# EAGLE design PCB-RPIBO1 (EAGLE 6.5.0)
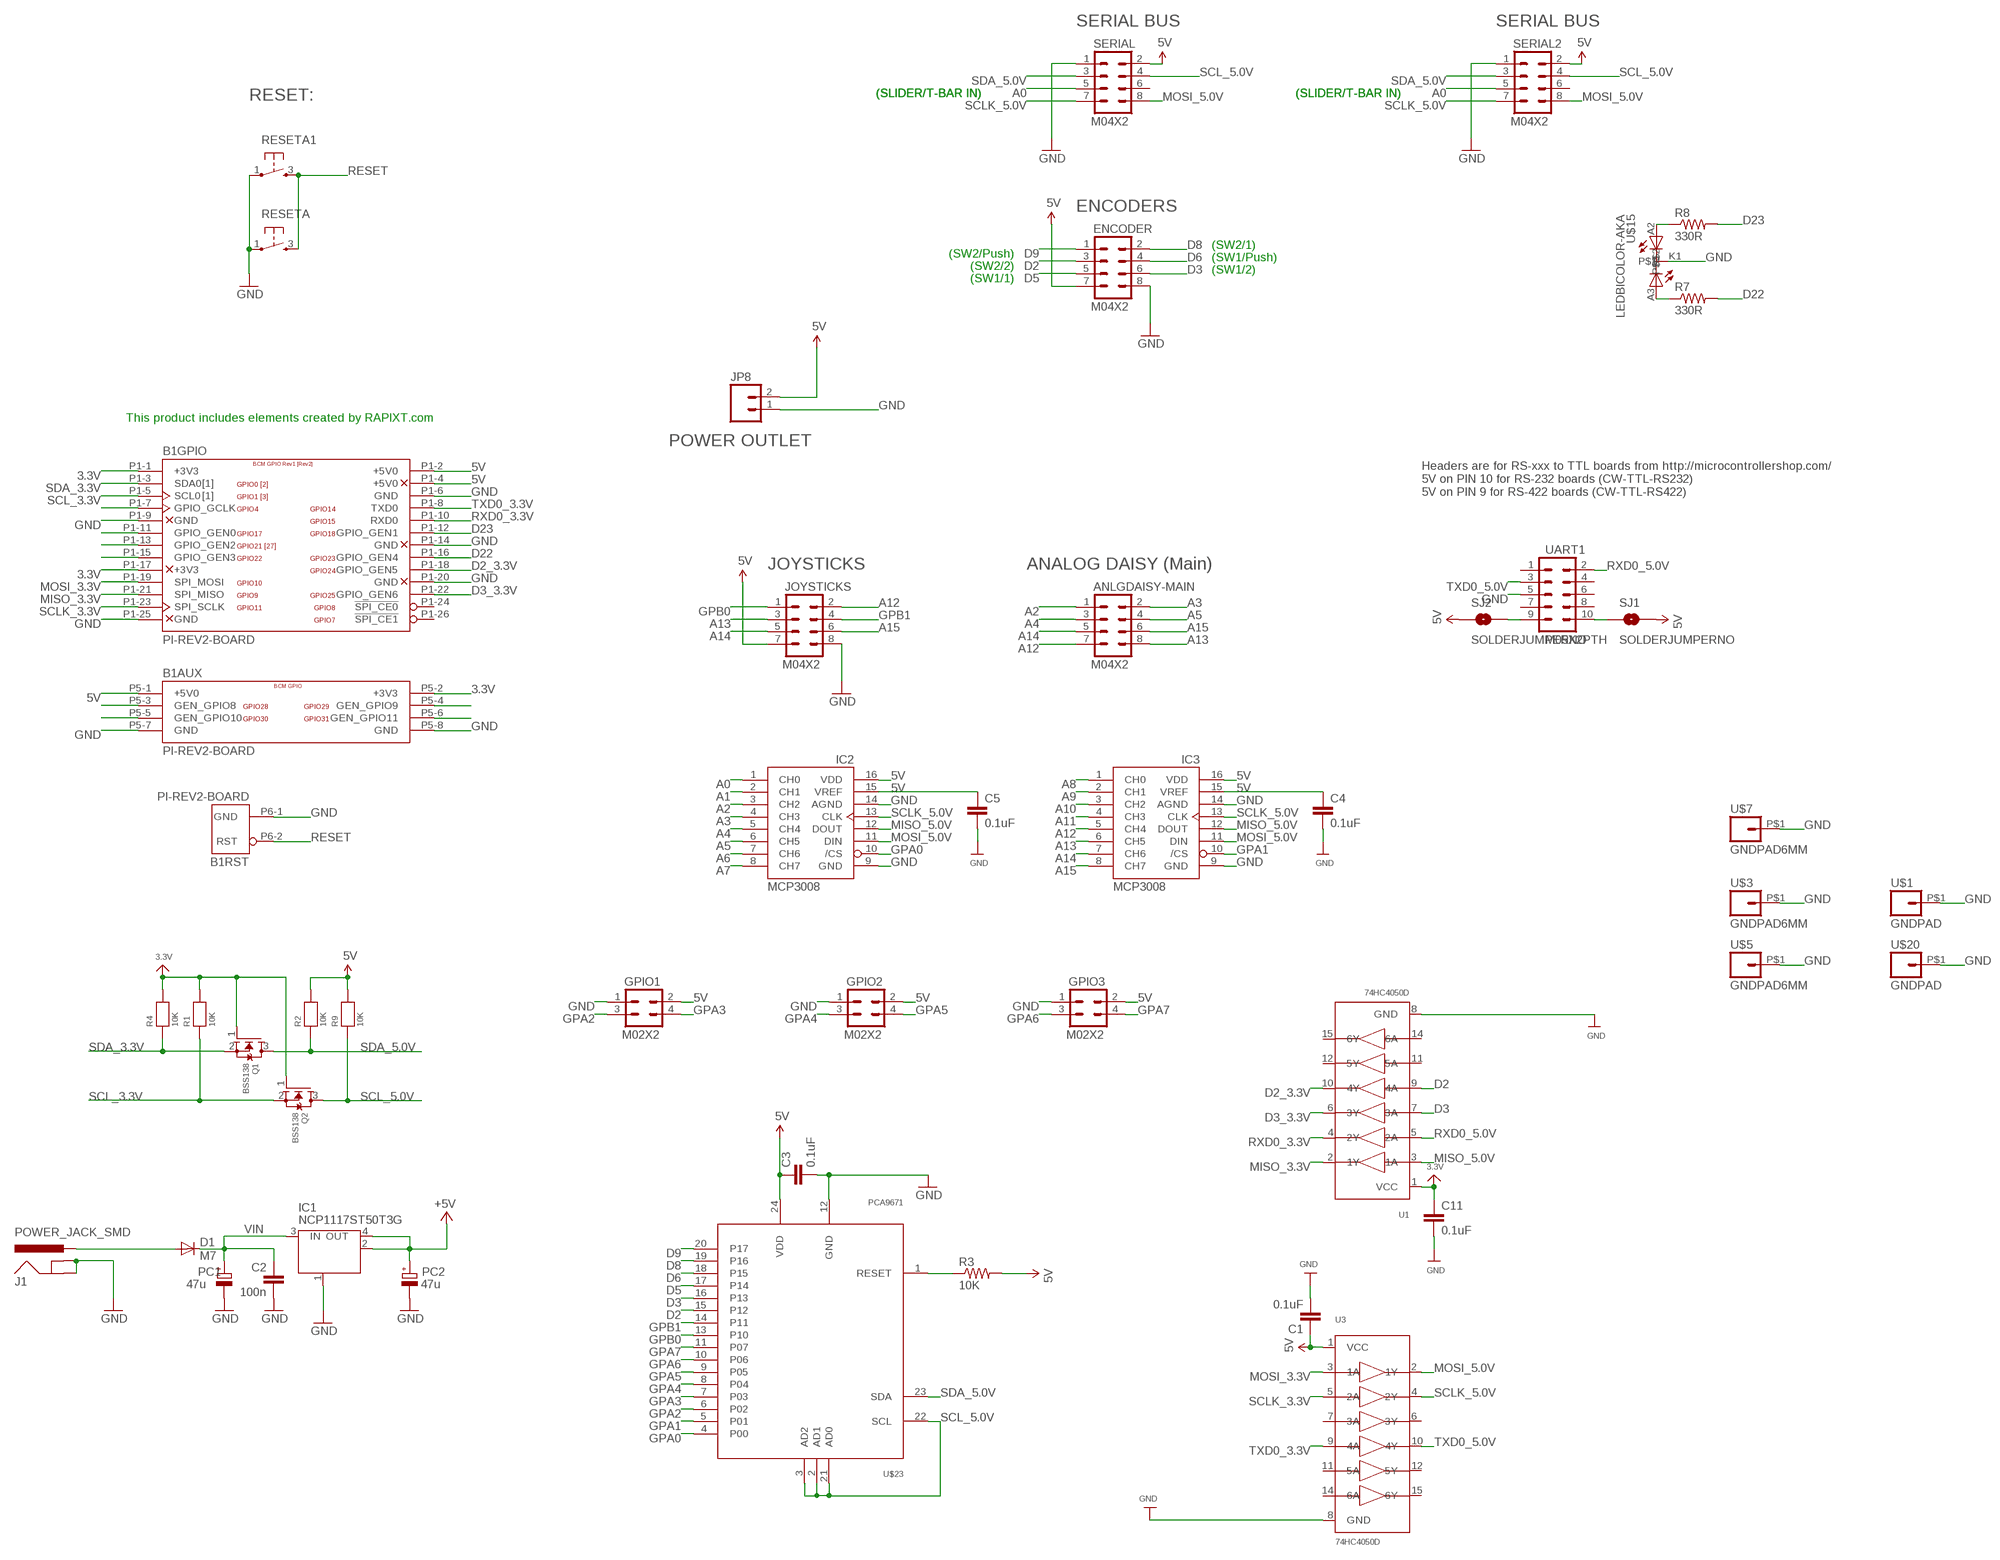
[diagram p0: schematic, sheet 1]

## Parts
ANLGDAISY-MAIN  M04X2  [2X4]
B1  PI-REV2-BOARD  [RASPBERRY-PI-REV2]
C1  0.1uF  CAP0603-CAP  [0603-CAP]
C2  100n  C-EU0603-RND  [C0603-ROUND]
C3  0.1uF  CAP0603-CAP  [0603-CAP]
C4  0.1uF  CAP0603-CAP  [0603-CAP]
C5  0.1uF  CAP0603-CAP  [0603-CAP]
C11  0.1uF  CAP0603-CAP  [0603-CAP]
D1  M7  DIODE-SMB  [SMB]
ENCODER  M04X2  [2X4]
GPIO1  M02X2  [2X2]
GPIO2  M02X2  [2X2]
GPIO3  M02X2  [2X2]
IC1  NCP1117ST50T3G  MC33269ST-3.3T3  [SOT223]
IC2  MCP3008  [DIL16]
IC3  MCP3008  [DIL16]
J1  POWER_JACK_SMD  [POWER_JACK_SMD]
JOYSTICKS  M04X2  [2X4]
JP8  M02PTH4  [1X02_XTRA_BIG]
PC1  47u  CPOL-EUD  [PANASONIC_D]
PC2  47u  CPOL-EUD  [PANASONIC_D]
Q1  BSS138  MOSFET-NWIDE  [SOT23-WIDE]
Q2  BSS138  MOSFET-NWIDE  [SOT23-WIDE]
R1  10K  RESISTOR0805  [0805]
R2  10K  RESISTOR0805  [0805]
R3  10K  RESISTOR0603-RES  [0603-RES]
R4  10K  RESISTOR0805  [0805]
R7  330R  RESISTOR0603-RES  [0603-RES]
R8  330R  RESISTOR0603-RES  [0603-RES]
R9  10K  RESISTOR0805  [0805]
RESETA  TAC_SWITCH  [PUSHBUTTON]
RESETA1  TAC_SWITCH  [PUSHBUTTON]
SERIAL  M04X2  [2X4]
SERIAL2  M04X2  [2X4]
SJ1  SOLDERJUMPERNO  [SJ_2S-NO]
SJ2  SOLDERJUMPERNO  [SJ_2S-NO]
U1  74HC4050D  [SOIC16]
U3  74HC4050D  [SOIC16]
U$1  GNDPAD  [3.2MMPAD]
U$3  GNDPAD6MM  [3.2MMPAD6MM]
U$5  GNDPAD6MM  [3.2MMPAD6MM]
U$7  GNDPAD6MM  [3.2MMPAD6MM]
U$15  LEDBICOLOR-AKA  [LED5MM-BICOLOR]
U$20  GNDPAD  [3.2MMPAD]
U$23  PCA9671  [TSSOP24]
UART1  M05X2PTH  [AVR_ICSP]

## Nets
3.3V [Power]: B1.P1-1(GPIO:+3V3) B1.P1-17(GPIO:+3V3) B1.P5-2(AUX:+3V3) C11.1 Q1.1(G) Q2.1(G) R1.2 R4.2 U1.1(VCC)
5V [Power]: B1.P1-2(GPIO:+5V0) B1.P1-4(GPIO:+5V0) B1.P5-1(AUX:+5V0) C1.1 C3.1 C4.1 C5.1 ENCODER.7 GPIO1.2 GPIO2.2 GPIO3.2 IC1.2(OUT) IC1.4(OUT) IC2.15(VREF) IC2.16(VDD) IC3.15(VREF) IC3.16(VDD) JOYSTICKS.7 JP8.2 PC2.+ R2.2 R3.2 R9.2 SERIAL2.2 SERIAL.2 SJ1.2 SJ2.1 U3.1(VCC) U$23.24(VDD) ; supply symbol labelled +5V
12V [Power]: D1.A J1.PWR
A0: IC2.1(CH0) SERIAL2.5 SERIAL.5
A1: IC2.2(CH1)
A2: ANLGDAISY-MAIN.1 IC2.3(CH2)
A3: ANLGDAISY-MAIN.2 IC2.4(CH3)
A4: ANLGDAISY-MAIN.3 IC2.5(CH4)
A5: ANLGDAISY-MAIN.4 IC2.6(CH5)
A6: IC2.7(CH6)
A7: IC2.8(CH7)
A8: IC3.1(CH0)
A9: IC3.2(CH1)
A10: IC3.3(CH2)
A11: IC3.4(CH3)
A12: ANLGDAISY-MAIN.7 IC3.5(CH4) JOYSTICKS.2
A13: ANLGDAISY-MAIN.8 IC3.6(CH5) JOYSTICKS.3
A14: ANLGDAISY-MAIN.5 IC3.7(CH6) JOYSTICKS.5
A15: ANLGDAISY-MAIN.6 IC3.8(CH7) JOYSTICKS.6
D2: ENCODER.3 U1.9(4A) U$23.15(P12)
D2_3.3V: B1.P1-18(GPIO:GPIO_GEN5) U1.10(4Y)
D3: ENCODER.6 U1.7(3A) U$23.16(P13)
D3_3.3V: B1.P1-22(GPIO:GPIO_GEN6) U1.6(3Y)
D5: ENCODER.5 U$23.17(P14)
D6: ENCODER.4 U$23.18(P15)
D8: ENCODER.2 U$23.19(P16)
D9: ENCODER.1 U$23.20(P17)
D22: B1.P1-16(GPIO:GPIO_GEN4) R7.2
D23: B1.P1-12(GPIO:GPIO_GEN1) R8.2
GND [Power]: B1.P1-6(GPIO:GND) B1.P1-9(GPIO:GND) B1.P1-14(GPIO:GND) B1.P1-20(GPIO:GND) B1.P1-25(GPIO:GND) B1.P5-7(AUX:GND) B1.P5-8(AUX:GND) B1.P6-1(RST:GND) C1.2 C2.2 C3.2 C4.2 C5.2 C11.2 ENCODER.8 GPIO1.1 GPIO2.1 GPIO3.1 IC1.1(GND/ADJ) IC2.9(GND) IC2.14(AGND) IC3.9(GND) IC3.14(AGND) J1.GND J1.SHUNT(GNDBREAK) JOYSTICKS.8 JP8.1 PC1.- PC2.- RESETA1.1 RESETA.1 SERIAL2.1 SERIAL.1 U1.8(GND) U3.8(GND) U$1.P$1 U$3.P$1 U$5.P$1 U$7.P$1 U$15.K1 U$20.P$1 U$23.12(GND) UART1.5
GPA0: IC2.10(/CS) U$23.4(P00)
GPA1: IC3.10(/CS) U$23.5(P01)
GPA2: GPIO1.3 U$23.6(P02)
GPA3: GPIO1.4 U$23.7(P03)
GPA4: GPIO2.3 U$23.8(P04)
GPA5: GPIO2.4 U$23.9(P05)
GPA6: GPIO3.3 U$23.10(P06)
GPA7: GPIO3.4 U$23.11(P07)
GPB0: JOYSTICKS.1 U$23.13(P10)
GPB1: JOYSTICKS.4 U$23.14(P11)
MISO_3.3V: B1.P1-21(GPIO:SPI_MISO) U1.2(1Y)
MISO_5.0V: IC2.12(DOUT) IC3.12(DOUT) U1.3(1A)
MOSI_3.3V: B1.P1-19(GPIO:SPI_MOSI) U3.3(1A)
MOSI_5.0V: IC2.11(DIN) IC3.11(DIN) SERIAL2.8 SERIAL.8 U3.2(1Y)
N$1: R3.1 U$23.1(RESET)
N$9: SJ2.2 UART1.9
N$10: SJ1.1 UART1.10
N$17: R8.1 U$15.A2
N$22: R7.1 U$15.A3
N$23: B1.P1-15(GPIO:GPIO_GEN3)
N$24: B1.P1-13(GPIO:GPIO_GEN2)
N$25: B1.P1-11(GPIO:GPIO_GEN0)
N$27: B1.P1-7(GPIO:GPIO_GCLK)
N$34: B1.P5-4(AUX:GEN_GPIO9)
N$35: B1.P5-6(AUX:GEN_GPIO11)
N$38: B1.P5-3(AUX:GEN_GPIO8)
N$39: B1.P5-5(AUX:GEN_GPIO10)
RESET: B1.P6-2(RST:RST) RESETA1.3 RESETA.3
RXD0_3.3V: B1.P1-10(GPIO:RXD0) U1.4(2Y)
RXD0_5.0V: U1.5(2A) UART1.2
SCL_3.3V: B1.P1-5(GPIO:SCL0) Q2.2(S) R1.1
SCL_5.0V: Q2.3(D) R9.1 SERIAL2.4 SERIAL.4 U$23.2(AD1) U$23.3(AD2) U$23.21(AD0) U$23.22(SCL)
SCLK_3.3V: B1.P1-23(GPIO:SPI_SCLK) U3.5(2A)
SCLK_5.0V: IC2.13(CLK) IC3.13(CLK) SERIAL2.7 SERIAL.7 U3.4(2Y)
SDA_3.3V: B1.P1-3(GPIO:SDA0) Q1.2(S) R4.1
SDA_5.0V: Q1.3(D) R2.1 SERIAL2.3 SERIAL.3 U$23.23(SDA)
TXD0_3.3V: B1.P1-8(GPIO:TXD0) U3.9(4A)
TXD0_5.0V: U3.10(4Y) UART1.3
VIN [Power]: C2.1 D1.C IC1.3(IN) PC1.+
Unconnected: B1.P1-24(GPIO:!SPI_CE0) B1.P1-26(GPIO:!SPI_CE1) SERIAL2.6 SERIAL.6 U1.11(5A) U1.12(5Y) U1.14(6A) U1.15(6Y) U3.6(3Y) U3.7(3A) U3.11(5A) U3.12(5Y) U3.14(6A) U3.15(6Y) UART1.1 UART1.4 UART1.6 UART1.7 UART1.8

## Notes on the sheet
- SERIAL BUS | SERIAL BUS
- (SLIDER/T-BAR IN) | (SLIDER/T-BAR IN) | (SLIDER/T-BAR IN) | (SLIDER/T-BAR IN)
- RESET:
- ENCODERS
- (SW2/Push) | (SW2/1)
- (SW2/2) | (SW1/Push)
- (SW1/1) | (SW1/2)
- This product includes elements created by RAPIXT.com
- POWER OUTLET
- Headers are for RS-xxx to TTL boards from http://microcontrollershop.com/
  5V on PIN 10 for RS-232 boards (CW-TTL-RS232)
  5V on PIN 9 for RS-422 boards (CW-TTL-RS422)
- JOYSTICKS | ANALOG DAISY (Main)

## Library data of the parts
ANLGDAISY-MAIN ENCODER JOYSTICKS SERIAL SERIAL2 = SparkFun:M04X2
B1 = SKAARHOJ:PI-REV2-: Raspberry Pi Rev2
C1 C3-C5 C11 = SparkFun:CAP: Capacitor
C2 = SmartPrj:C-EU: CAPACITOR, European symbol
D1 = diode:DIODE-: DIODE
GPIO1-GPIO3 = SKAARHOJ:M02X2
IC1 = linear:MC33269ST*: Adjustable Output Low Dropout Voltage Regulator 800 mA Source: http://www.onsemi.com/pub/Collateral/MC33269-D.PDF
IC2 IC3 = adafruit:MCP3008
J1 = SKAARHOJ:POWER_JACK_SMD: RASM712PX Right Angle SMT Mount DC Power Jack, pin size 0.100"(2.5mm), with locating post Switchcraft.com
JP8 = SparkFun:M02: Header 2
PC1 PC2 = rcl:CPOL-EU: POLARIZED CAPACITOR, European symbol
Q1 Q2 = microbuilder:MOSFET-N: N-Channel Mosfet LEGEND VDS: Voltage Drain-Source ID: Drain Current RDS(ON): Drain-Source On-State Resistance VGS(TH): Gate-Source Threshold Voltage CISS: Drain-Source Input Capacitance SOT-23 Name VDS ID RDS(ON) VGS(TH) CISS Order Number 2N7002E 60V 260mA 2.5 Ohm 2.5V @ 250uA 26.7pF @ 25V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
R1 R2 R4 R9 = microbuilder:RESISTOR: Resistors
R3 R7 R8 = SparkFun:RESISTOR: Resistor
RESETA RESETA1 = SKAARHOJ:TAC_SWITCH: Momentary Switch
SJ1 SJ2 = SparkFun:SOLDERJUMPER: Solder Jumper
U1 U3 = microbuilder:74HC4050D: 6-channel level shifter 74HC4050D - 2V-6V Supply Digikey: 74HC4050D,653-ND Mouser: 771-74HC4050D-T
U$1 U$3 U$5 U$7 U$20 = SKAARHOJ:GNDPAD
U$15 = SKAARHOJ:LEDBICOLOR-AKA
U$23 = SKAARHOJ:PCA9671
UART1 = SparkFun:M05X2: Header 5x2 Standard 10-pin dual row 0.1" header. Commonly used with AVR-ISP. Use with Spark Fun Electronics SKU: PRT-00778

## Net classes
0 default: width 0.203 mm, drill 0.406 mm, clearance 0.152 mm
1 Power: width 0.508 mm, drill 0.61 mm, clearance 0.203 mm
3 INput lines: clearance 0.203 mm

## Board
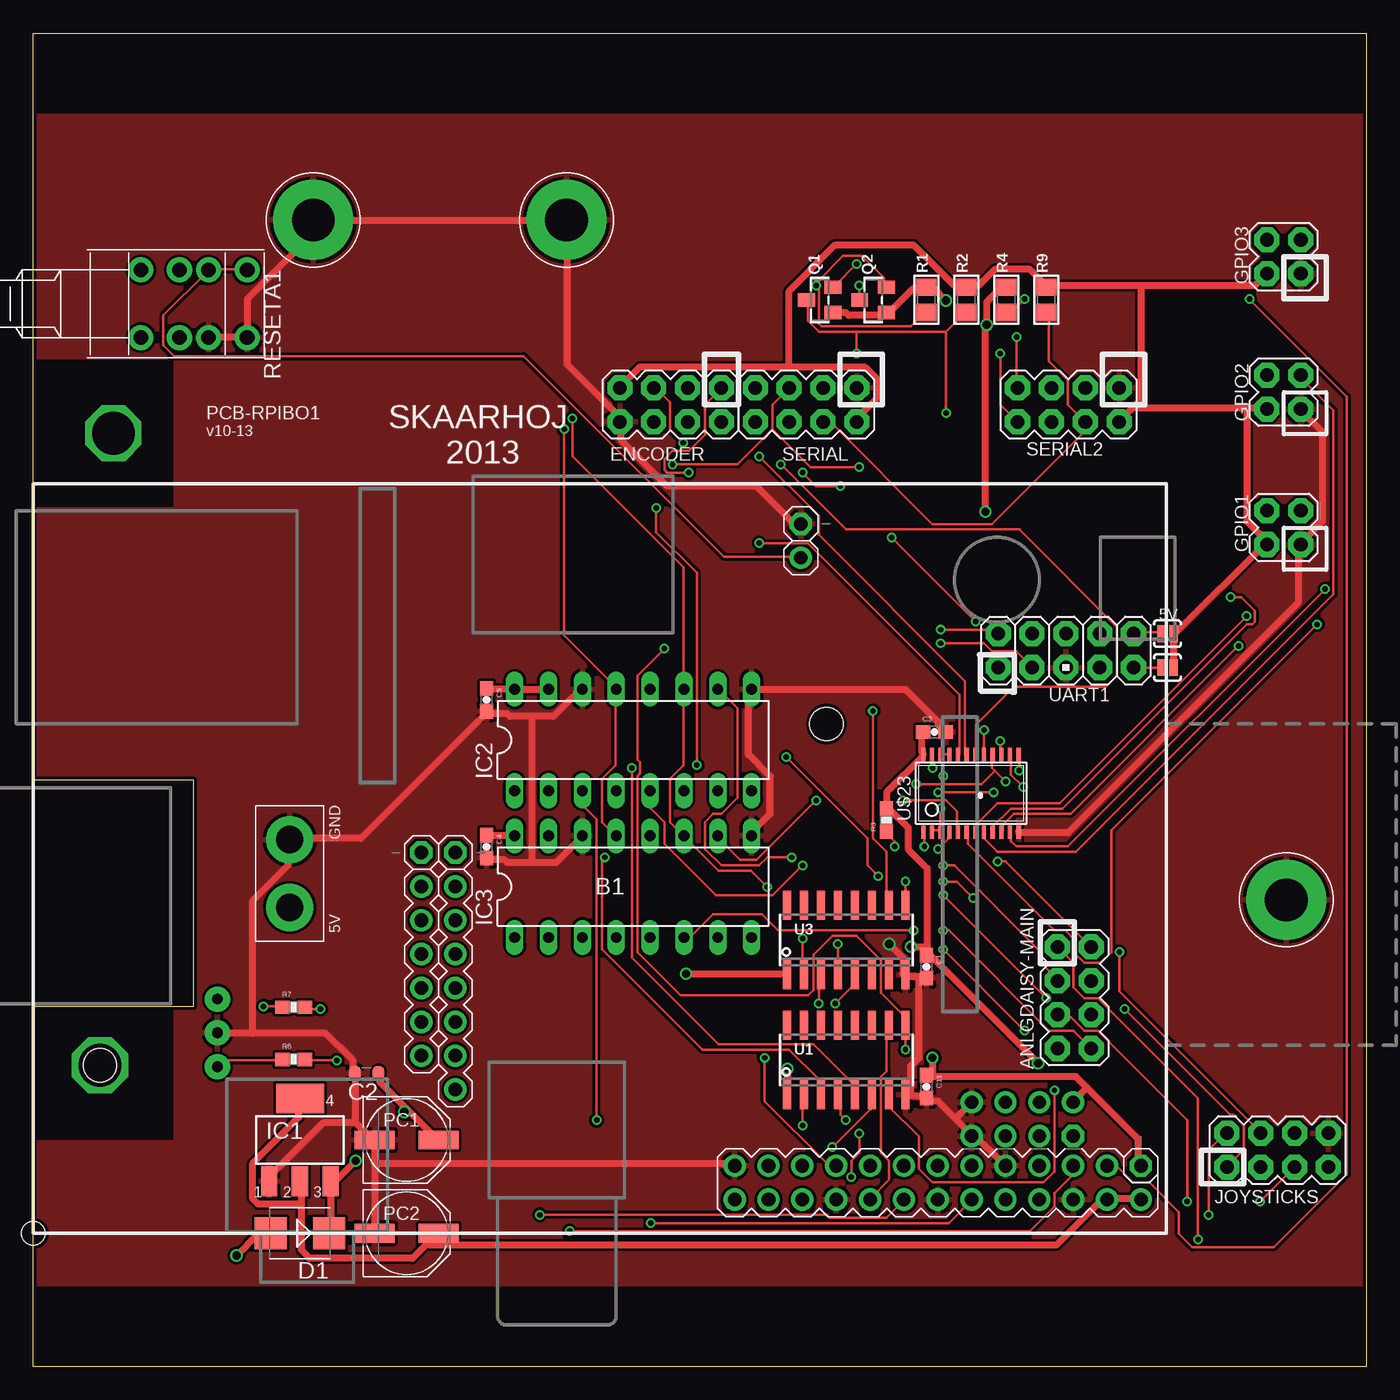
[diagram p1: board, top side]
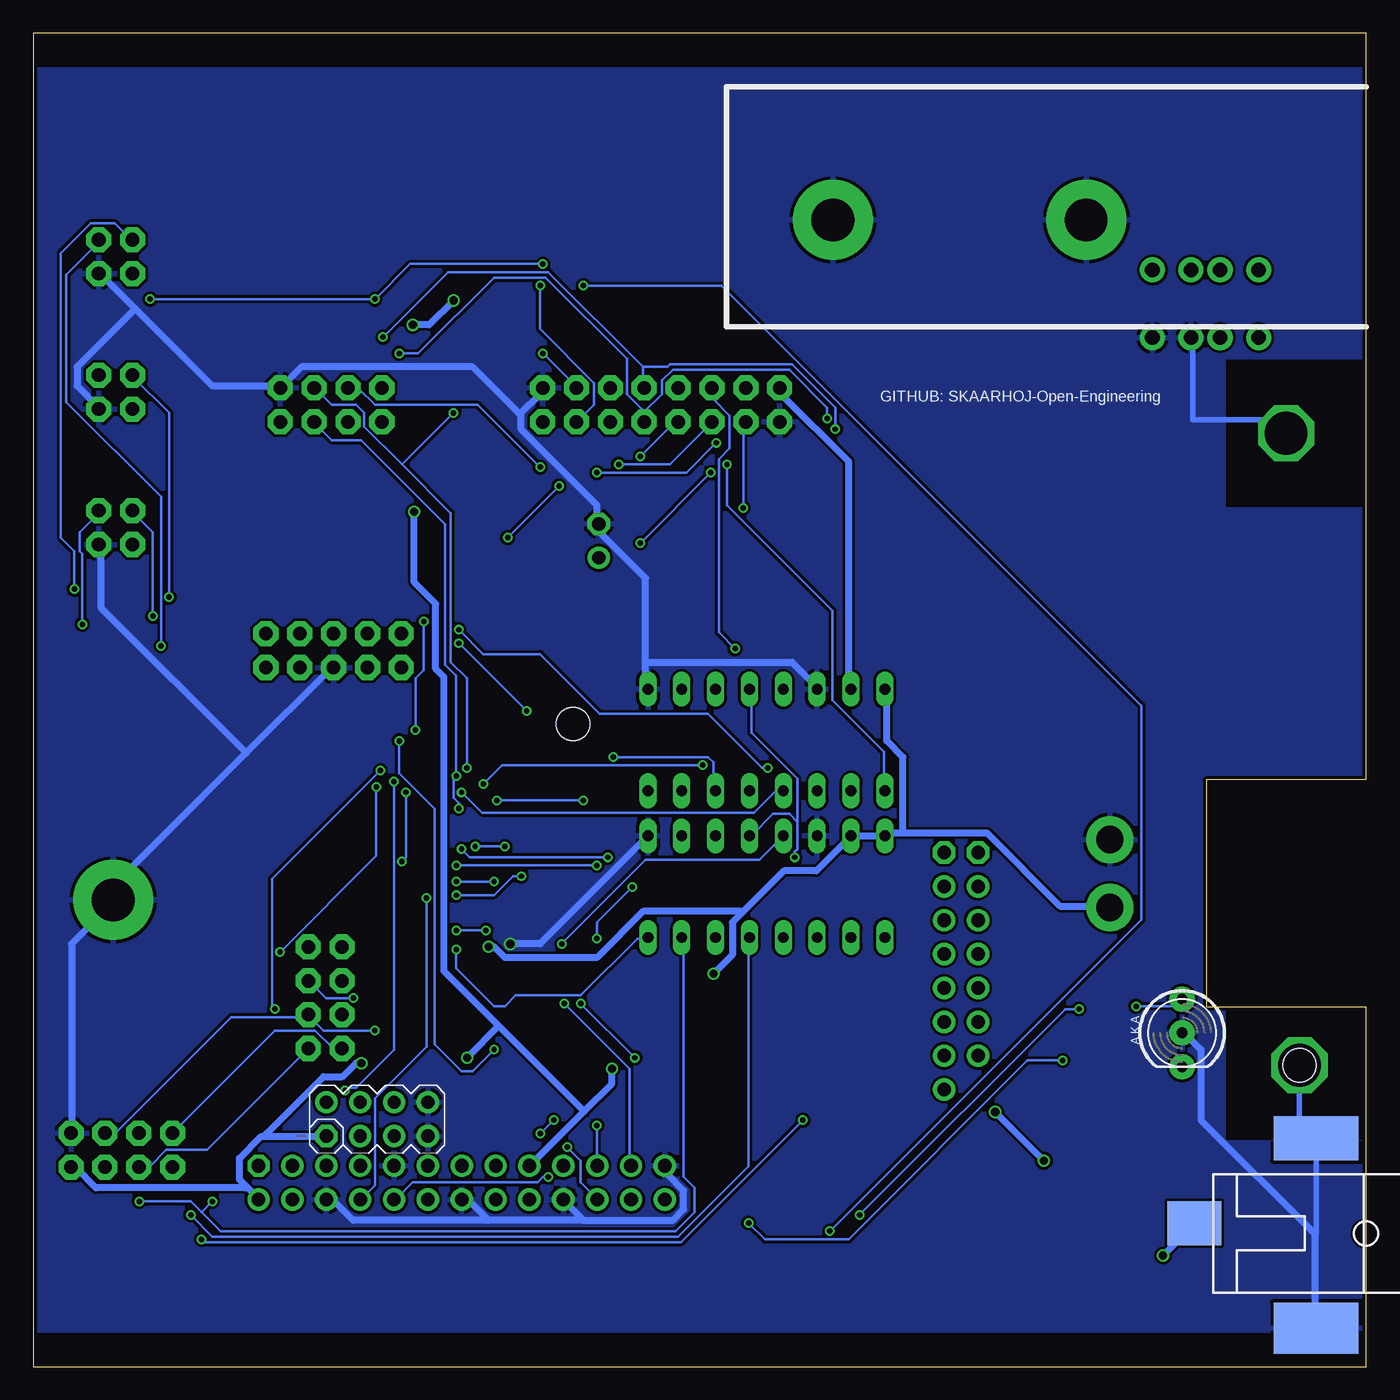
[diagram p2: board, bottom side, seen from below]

Size 100 x 100 mm. Coordinates in mm from the lower left corner, seen from the top.
Outline: 0,0 0,27 12,27 12,44 0,44 0,100 100,100 100,0 0,0
Copper layers (1*16): Top 0.035mm / dielectric 1.5mm / Bottom 0.035mm
Design rules "Fusion_eagle_rule_v1.1": minimum track width 6mil, minimum drill 12mil, track to track 6mil, track to pad 6mil, pad to pad 6mil, via to via 6mil, smd to smd 0mil, copper to edge 10mil, drill to drill 10mil, minimum pad ring 10mil, minimum via ring 6mil, stop-mask expansion 2mil, vias tented up to drill 100mil, thermal gap 10mil
tRestrict: area 0,17 to 10.5,28; area 0,64.5 to 10.5,75.5; area 0,94 to 100,100; area 0,0 to 100,6
bRestrict: area 0,64.5 to 10.5,75.5; area 0,17 to 10.5,28; area 0,0 to 100,2.5; area 0,97.5 to 100,100

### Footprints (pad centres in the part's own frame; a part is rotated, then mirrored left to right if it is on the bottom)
2X4 = drill 1.016 pad 1.88 octagon: 1 -3.81,-1.27; 2 -3.81,1.27; 3 -1.27,-1.27; 4 -1.27,1.27; 5 1.27,-1.27; 6 1.27,1.27; 7 3.81,-1.27; 8 3.81,1.27
RASPBERRY-PI-REV2 = drill 1.016 pad 1.676 octagon: P1-1 83.095,5.065; P2-1 31.66,28.56; P3-1 29.12,28.56 | drill 1.016 pad 1.676: P1-2 83.095,2.525; P1-3 80.555,5.065; P1-4 80.555,2.525; P1-5 78.015,5.065; P1-6 78.015,2.525; P1-7 75.475,5.065; P1-8 75.475,2.525; P1-9 72.935,5.065; P1-10 72.935,2.525; P1-11 70.395,5.065; P1-12 70.395,2.525; P1-13 67.855,5.065; P1-14 67.855,2.525; P1-15 65.315,5.065; P1-16 65.315,2.525; P1-17 62.775,5.065; P1-18 62.775,2.525; P1-19 60.235,5.065; P1-20 60.235,2.525; P1-21 57.695,5.065; P1-22 57.695,2.525; P1-23 55.155,5.065; P1-24 55.155,2.525; P1-25 52.615,5.065; P1-26 52.615,2.525; P2-2 31.66,26.02; P2-3 31.66,23.48; P2-4 31.66,20.94; P2-5 31.66,18.4; P2-6 31.66,15.86; P2-7 31.66,13.32; P2-8 31.66,10.78; P3-2 29.12,26.02; P3-3 29.12,23.48; P3-4 29.12,20.94; P3-5 29.12,18.4; P3-6 29.12,15.86; P3-7 29.12,13.32 | drill 1 pad 1.676 octagon: P5-1 78.015,7.287; P6-1 57.58,53.21 | drill 1 pad 1.676: P5-2 78.015,9.828; P5-3 75.475,7.287; P5-4 75.475,9.828; P5-5 72.935,7.287; P5-6 72.935,9.828; P5-7 70.395,7.287; P5-8 70.395,9.828; P6-2 57.58,50.67 | hole 2.5: 59.5,38.2; 5,12.6
0603-CAP = smd 1.1 x 1: 1 -0.85,0; 2 0.85,0
C0603-ROUND = smd 0.898 x 1.1: 1 -0.889,0; 2 0.889,0
SMB = smd 2.4 x 2.4: A 2.2,0; C -2.2,0
2X2 = drill 1.016 pad 1.88 octagon: 1 -3.81,-1.27; 2 -3.81,1.27; 3 -1.27,-1.27; 4 -1.27,1.27
SOT223 = smd 1.219 x 2.235: 1 -2.311,-3.099; 2 0,-3.099; 3 2.311,-3.099 | smd 3.6 x 2.2: 4 0,3.099
DIL16 = drill 0.813 long: 1 -8.89,-3.81; 2 -6.35,-3.81; 3 -3.81,-3.81; 4 -1.27,-3.81; 5 1.27,-3.81; 6 3.81,-3.81; 7 6.35,-3.81; 8 8.89,-3.81; 9 8.89,3.81; 10 6.35,3.81; 11 3.81,3.81; 12 1.27,3.81; 13 -1.27,3.81; 14 -3.81,3.81; 15 -6.35,3.81; 16 -8.89,3.81
POWER_JACK_SMD = smd 6.35 x 3.81: GND -6.756,-7.112 | smd 4.064 x 3.302: PWR -15.9,0.762 | smd 6.35 x 3.302: SHUNT -6.756,7.112 | hole 1.778: -2.997,0
1X02_XTRA_BIG = drill 2.057 pad 3.556: 1 -2.54,0; 2 2.54,0
PANASONIC_D = smd 3 x 1.4: + 2.4,0; - -2.4,0
SOT23-WIDE = smd 1 x 1.27: 1 -0.95,-1; 2 0.95,-1; 3 0,1
0805 = smd 1.3 x 1.5: 1 -0.95,0; 2 0.95,0
0603-RES = smd 1.1 x 1: 1 -0.85,0; 2 0.85,0
PUSHBUTTON = drill 1.1 pad 1.88: 1 2.54,2.54; 2 2.54,-2.54; 3 -2.54,2.54; 4 -2.54,-2.54
SJ_2S-NO = smd 0.635 x 1.27: 1 -0.45,0; 2 0.45,0
SOIC16 = smd 0.6 x 2.2: 1 -4.445,-2.6; 2 -3.175,-2.6; 3 -1.905,-2.6; 4 -0.635,-2.6; 5 0.635,-2.6; 6 1.905,-2.6; 7 3.175,-2.6; 8 4.445,-2.6; 9 4.445,2.6; 10 3.175,2.6; 11 1.905,2.6; 12 0.635,2.6; 13 -0.635,2.6; 14 -1.905,2.6; 15 -3.175,2.6; 16 -4.445,2.6
3.2MMPAD = drill 3.2 octagon: P$1 0,0
3.2MMPAD6MM = drill 3.2 pad 6: P$1 0,0
LED5MM-BICOLOR = drill 0.813 pad 1.88: A2 2.54,0; A3 -2.54,0; K1 0,0
TSSOP24 = smd 0.305 x 0.991: 1 -4.225,-2.918; 2 -3.575,-2.918; 3 -2.925,-2.918; 4 -2.275,-2.918; 5 -1.625,-2.918; 6 -0.975,-2.918; 7 -0.325,-2.918; 8 0.325,-2.918; 9 0.975,-2.918; 10 1.625,-2.918; 11 2.275,-2.918; 12 2.925,-2.918; 13 2.925,2.918; 14 2.275,2.918; 15 1.625,2.918; 16 0.975,2.918; 17 0.325,2.918; 18 -0.325,2.918; 19 -0.975,2.918; 20 -1.625,2.918; 21 -2.275,2.918; 22 -2.925,2.918; 23 -3.575,2.918; 24 -4.225,2.918
AVR_ICSP = drill 1.016 pad 1.88 octagon: 1 -1.27,5.08; 2 1.27,5.08; 3 -1.27,2.54; 4 1.27,2.54; 5 -1.27,0; 6 1.27,0; 7 -1.27,-2.54; 8 1.27,-2.54; 9 -1.27,-5.08; 10 1.27,-5.08

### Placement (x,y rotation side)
ANLGDAISY-MAIN  78.11,27.67 270 top
B1  0,10 0 top
C1  67,30 270 top
C2  25,22 180 top
C3  67.6,47.6 0 top
C4  34,39 270 top
C5  34,50 270 top
C11  67,21 270 top
D1  20,10 180 top
ENCODER  47.81,72.14 180 top
GPIO1  93.83,65.47 90 top
GPIO2  93.83,75.63 90 top
GPIO3  93.83,85.79 90 top
IC1  20,17 0 top
IC2  45,47 0 top
IC3  45,36 0 top
J1  -3,10 0 bottom
JOYSTICKS  93.36,16.24 0 top
JP8  19.23,36.98 270 top
PC1  28,17 0 top
PC2  28,10 0 top
Q1  59,80 90 top
Q2  63,80 90 top
R1  67,80 90 top
R2  70,80 90 top
R3  64,41 90 top
R4  73,80 90 top
R7  19.52,26.95 0 top
R8  19.52,23.05 0 top
R9  76,80 90 top
RESETA  10.6,79.72 270 top
RESETA1  13.5,79.72 270 top
SERIAL  57.98,72.14 180 top
SERIAL2  77.66,72.14 180 top
SJ1  85.09,54.98 0 top
SJ2  85.09,52.44 180 top
U1  61,23 0 top
U3  61,32 0 top
U$1  6,70 0 top
U$3  21,86 0 top
U$5  40,86 0 top
U$7  94,35 0 top
U$15  13.81,25.03 270 bottom
U$20  5,22.6 0 top
U$23  71,43 0 top
UART1  77.47,53.7 90 top

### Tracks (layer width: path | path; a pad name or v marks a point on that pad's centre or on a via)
3.3V  (via drill 0.61)
  Top 0.508: 79.05,20.93 82.91,17.07 82.91,15.24 B1.P1-1 | 79.05,20.93 78.23,21.74 67.06,21.74 C11.1 67.46,21.95 v67.46,23.16 | Q1.1 60.15,79.05 60.96,79.05 61.16,78.84 63.6,78.84 63.8,79.05 Q2.1 64.21,79.05 66.04,80.87 66.85,80.87 R1.2 67.26,80.97 67.46,80.97 v68.48,79.96 | R4.2 72.95,80.87 72.54,80.87 71.53,79.86 v71.53,78.13 71.42,77.93 v71.42,64.11 | v56.59,22.35 56.59,20.42 U1.1 | 79.05,20.93 78.03,19.91 B1.P5-2
  Bottom 0.508: v71.53,78.13 70.31,78.13 v68.48,79.96 | v56.59,22.35 56.59,21.23 58.67,19.15 | 58.67,19.15 62.69,15.14 B1.P1-17 | v71.42,64.11 71.42,58.83 69.8,57.2 69.8,52.32 69.19,51.71 69.19,29.67 65.08,25.55 | 58.67,19.15 65.08,25.55 | 65.08,25.55 v67.46,23.16
5V  (via drill 0.61)
  Top 0.508: 67.06,31.5 67.06,37.39 65.63,38.81 65.63,40.44 64.21,41.86 R3.2 64.01,43.08 66.65,45.72 U$23.24 66.65,46.13 66.65,47.55 C3.1 | 67.06,31.5 67.06,30.89 C1.1 67.26,30.89 v75.39,22.76 | B1.P1-2 82.91,12.6 80.67,12.6 B1.P1-4 80.47,12.39 80.06,12.39 76.81,9.14 29.67,9.14 29.57,9.25 | SJ2.1 85.55,52.63 85.55,54.86 SJ1.2 85.75,55.07 92.46,61.77 GPIO1.2 92.46,61.98 91.03,63.4 91.03,71.93 | 83.11,81.08 91.64,81.08 92.46,81.89 GPIO3.2 | 83.11,81.08 76.2,81.08 R9.2 76,81.08 74.78,82.3 72.14,82.3 70.92,81.08 70.1,81.08 R2.2 69.9,81.08 69.09,81.08 66.04,84.12 60.15,84.12 56.69,80.67 56.69,74.98 | 82.6,72.03 83.11,72.54 83.11,81.08 | 82.6,72.03 81.48,70.92 SERIAL2.2 | 91.03,71.93 82.7,71.93 82.6,72.03 | 91.03,71.93 92.46,71.93 GPIO2.2 | C5.1 34.14,50.8 35.97,50.8 IC2.16 36.17,50.8 38.61,50.8 IC2.15 | 56.69,74.98 45.52,74.98 44.09,73.56 ENCODER.7 | 56.69,74.98 62.38,74.98 63.4,73.97 63.4,72.75 61.98,71.32 61.98,70.92 SERIAL.2 | 20.12,12.19 20.12,8.74 20.73,8.13 28.45,8.13 29.57,9.25 | 20.12,12.19 20.12,13.82 IC1.2 | 29.57,9.25 30.28,9.96 PC2.+ | 20.12,12.19 16.87,12.19 16.46,12.6 16.46,15.24 19.91,18.69 19.91,19.91 IC1.4 | C4.1 34.14,39.83 35.97,39.83 IC3.16 | v48.97,29.46 56.49,29.46 U3.1 | v65.84,31.5 67.06,31.5
  Bottom 0.508: 82.5,17.27 82.91,17.27 84.53,15.65 84.53,14.02 84.02,13.51 | 82.5,17.27 78.03,17.27 B1.P5-1 | 84.02,13.51 83.11,12.6 B1.P1-2 | JOYSTICKS.7 97.13,14.83 96.72,14.83 95.3,13.41 84.12,13.41 84.02,13.51 | v75.39,22.76 75.79,22.76 76.81,21.74 78.23,21.74 82.5,17.48 82.5,17.27 | ENCODER.7 43.89,73.36 43.89,72.95 38.81,67.87 38.81,51 IC2.15 | v48.97,29.46 47.55,30.89 47.55,33.33 46.84,34.04 | 46.84,34.04 43.69,37.19 41.25,37.19 38.81,39.62 IC3.15 38.41,39.83 36.17,39.83 IC3.16 35.97,40.03 34.75,40.03 | 34.75,40.03 28.45,40.03 22.96,34.54 19.3,34.54 JP8.2 | 34.75,40.03 34.75,45.72 35.97,46.94 35.97,50.8 IC2.16 | v65.84,31.5 65.43,31.5 64.62,30.68 57.71,30.68 54.25,34.14 46.94,34.14 46.84,34.04
12V  (via drill 0.61)
  Top 0.508: v15.24,8.33 16.87,9.96 17.68,9.96 D1.A
  Bottom 0.508: v15.24,8.33 13.01,10.57 J1.PWR
A0  (via drill 0.41)
  Top 0.203: v47.95,67.67 52.83,67.67 55.47,70.31 | 55.47,70.31 55.47,72.14 56.69,73.36 SERIAL.5 | v61.98,67.46 58.32,67.46 55.47,70.31
  Bottom 0.203: v47.95,67.67 47.95,64.62 40.03,56.69 40.03,49.99 36.17,46.13 36.17,43.28 IC2.1 | v61.98,67.46 66.65,72.14 74.37,72.14 75.59,73.36 76.2,73.36 SERIAL2.5
A2  (via drill 0.41)
  Top 0.203: v42.27,18.49 42.27,41.05 41.25,42.06 41.25,43.08 IC2.3 | v87.38,9.55 87.38,20.12 79.86,27.64 78.84,27.64 78.03,28.45 78.03,30.28 77.01,31.29 ANLGDAISY-MAIN.1
  Bottom 0.203: v42.27,18.49 51.41,9.35 87.17,9.35 v87.38,9.55
A3  (via drill 0.41)
  Top 0.203: v72.03,43.08 v67.87,43.08 | v72.34,37.9 72.95,37.9 79.35,31.5 ANLGDAISY-MAIN.2
  Bottom 0.203: v67.87,43.08 66.34,41.55 45.92,41.55 44.3,43.18 43.79,43.18 IC2.4 | v72.03,43.08 72.03,38.2 v72.34,37.9
A4  (via drill 0.41)
  Top 0.203: v57.71,37.59 55.47,35.36 51.21,35.36 47.35,39.22 47.35,40.84 46.33,41.86 46.33,43.08 IC2.5 | v68.28,37.59 69.09,37.59 75.59,31.09 75.59,30.28 76.81,29.06 ANLGDAISY-MAIN.3
  Bottom 0.203: v68.28,37.59 v57.71,37.59
A5  (via drill 0.41)
  Top 0.203: v56.49,45.72 62.59,39.62 62.59,37.59 v63.4,36.78 | v76,27.64 v68.28,35.36
  Bottom 0.203: v56.49,45.72 49.38,45.72 48.97,45.31 48.97,43.28 IC2.6 | v63.4,36.78 64.01,36.78 65.43,35.36 v68.28,35.36 | v76,27.64 78.03,27.64 79.25,28.85 ANLGDAISY-MAIN.4
A12  (via drill 0.41)
  Top 0.203: v88.19,11.38 88.19,16.26 89.41,17.48 JOYSTICKS.2
  Bottom 0.203: v88.19,11.38 86.56,9.75 51.61,9.75 46.33,15.04 46.33,32.11 IC3.5 | ANLGDAISY-MAIN.7 77.01,23.98 77.62,23.98 78.84,25.2 81.89,25.2 89.41,17.68 JOYSTICKS.2
A13  (via drill 0.41)
  Top 0.203: v66.04,32.72 55.88,32.72 54.66,33.93 51,33.93 49.38,32.31 48.97,32.31 IC3.6 | v68.28,32.72 68.68,32.72 76.2,25.2 78.03,25.2 79.25,23.98 ANLGDAISY-MAIN.8
  Bottom 0.203: v68.28,32.72 v66.04,32.72 | JOYSTICKS.3 92.05,15.04 91.24,15.04 90.02,16.26 86.97,16.26 79.45,23.77 ANLGDAISY-MAIN.8
A14  (via drill 0.41)
  Top 0.203: v92.05,12.39 94.49,14.83 JOYSTICKS.5 | v86.56,12.39 86.56,18.49 79.86,25.2 78.84,25.2 77.83,26.21 77.01,26.21 ANLGDAISY-MAIN.5
  Bottom 0.203: 87.38,11.58 88.19,12.39 v92.05,12.39 | 87.38,11.58 85.95,10.16 51.82,10.16 50.39,11.58 50.39,13.41 51.21,14.22 51.21,32.11 IC3.7 | 87.38,11.58 v86.56,12.39
A15  (via drill 0.41)
  Top 0.203: v74.37,25.2 v68.28,31.29
  Bottom 0.203: v68.28,31.29 68.28,29.87 65.43,27.03 64.62,27.03 63.8,27.84 58.93,27.84 54.66,32.11 54.05,32.11 IC3.8 | v74.37,25.2 78.23,25.2 79.25,26.21 ANLGDAISY-MAIN.6 79.45,26.21 85.14,26.21 93.67,17.68 94.49,17.68 JOYSTICKS.6
D2  (via drill 0.41)
  Top 0.203: v72.54,46.94 72.54,45.92 U$23.15 | v65.43,23.77 65.43,25.4 U1.9 65.43,26.21 63.6,28.04 63.6,30.48 61.77,32.31 59.94,32.31 58.52,30.89 58.52,28.25 58.12,27.84 48.56,27.84 45.31,31.09 45.31,44.3 45.52,44.5 45.52,45.31 45.31,45.52 45.31,51.82 v47.35,53.85
  Bottom 0.203: v72.54,46.94 72.54,44.5 69.9,41.86 69.9,24.18 67.87,22.15 67.06,22.15 v65.43,23.77 | v47.35,53.85 48.56,55.07 48.56,68.07 47.75,68.89 47.75,71.32 48.97,72.54 48.97,73.36 ENCODER.3
D2_3.3V
  Top 0.203: U1.10 64.01,25.4 64.01,22.15 63.6,21.74 63.6,16.05 64.21,15.44 64.21,14.02 62.79,12.6 B1.P1-18
D3  (via drill 0.41)
  Top 0.203: v72.95,43.89 72.14,44.7 | 72.14,44.7 71.93,44.91 71.93,45.72 U$23.16 | v76.61,20.73 76.61,14.63 75.79,13.82 67.46,13.82 66.45,14.83 66.45,17.27 64.21,19.51 64.21,20.32 U1.7 | v46.74,64.41 46.74,62.59 49.78,59.54 v49.78,45.11 | v66.24,43.69 71.12,43.69 72.14,44.7
  Bottom 0.203: v72.95,43.89 72.95,23.77 75.79,20.93 76.4,20.93 v76.61,20.73 | v46.74,64.41 46.74,70.71 ENCODER.6 | v49.78,45.11 64.82,45.11 v66.24,43.69
D3_3.3V  (via drill 0.41)
  Top 0.203: v59.94,16.46 62.79,19.3 62.79,20.32 U1.6
  Bottom 0.203: v59.94,16.46 58.93,15.44 58.93,13.82 57.71,12.6 B1.P1-22
D5  (via drill 0.41)
  Top 0.203: v71.32,47.75 U$23.17 | v64.41,62.18 v70.71,55.88 | v60.55,66.04 58.73,66.04 v57.71,67.06 | v48.77,69.29 47.75,70.31 47.75,72.34 46.74,73.36 ENCODER.5
  Bottom 0.203: v71.32,47.75 71.32,51.61 70.71,52.22 v70.71,55.88 | v60.55,66.04 v64.41,62.18 | v57.71,67.06 51,67.06 v48.77,69.29
D6  (via drill 0.41)
  Top 0.203: v56.08,67.67 60.96,62.79 73.97,62.79 81.28,55.47 81.28,51.82 80.47,51 73.56,51 70.71,48.16 70.71,45.92 U$23.18
  Bottom 0.203: v56.08,67.67 52.22,67.67 49.17,70.71 ENCODER.4
D8  (via drill 0.41)
  Top 0.203: v54.46,68.28 58.93,63.8 58.93,62.38 69.9,51.41 69.9,45.92 U$23.19
  Bottom 0.203: v54.46,68.28 51.82,70.92 ENCODER.2
D9  (via drill 0.41)
  Top 0.203: v54.46,61.77 58.12,61.77 69.49,50.39 69.49,45.92 U$23.20 | v49.17,67.06 47.55,67.06 47.35,67.26 47.35,68.07 47.95,68.68 49.17,68.68 50.39,69.9 50.39,72.14 51.61,73.36 ENCODER.1
  Bottom 0.203: v49.17,67.06 v54.46,61.77
D22  (via drill 0.41)
  Top 0.203: v21.54,26.82 20.52,26.82 R7.2 | v38,11.38 59.54,11.38 59.74,11.18 64.01,11.18 65.23,12.39 B1.P1-16
  Bottom 0.203: v21.54,26.82 22.55,26.82 v38,11.38
D23  (via drill 0.41)
  Top 0.203: v22.76,22.96 20.52,22.96 R8.2 | v46.33,10.77 68.68,10.77 70.31,12.39 B1.P1-12
  Bottom 0.203: v22.76,22.96 25.4,22.96 38.81,9.55 45.11,9.55 v46.33,10.77
GND  (via drill 0.61)
  Top 0.508: 24.18,18.29 24.18,21.95 C2.2 23.98,22.15 23.98,22.96 21.95,24.99 16.46,24.99 | 24.18,18.29 25.4,17.07 PC1.- 25.6,16.87 25.6,15.24 | 24.18,18.29 21.74,18.29 17.88,14.43 17.88,14.02 IC1.1 | 25.6,15.24 25.6,10.16 PC2.- | 25.6,15.24 52.43,15.24 B1.P1-25 | GPIO2.1 95.1,71.73 96.72,70.1 96.72,63.4 95.1,61.77 GPIO1.1 94.89,61.57 94.89,57.3 77.62,40.03 73.97,40.03 U$23.12 | RESETA.1 13.21,77.22 15.85,77.22 RESETA1.1 16.05,77.42 16.05,80.06 20.93,84.94 20.93,85.95 U$3.P$1 21.13,85.95 39.83,85.95 U$5.P$1 40.03,85.95 40.03,75.18 43.89,71.32 43.89,70.92 ENCODER.8 44.09,70.71 44.09,69.49 47.55,66.04 54.25,66.04 56.9,63.4 57.51,63.4 B1.P6-1 | 66.45,29.26 65.63,29.26 U3.8 65.23,29.46 65.23,30.68 v64.21,31.7 | 66.45,29.26 66.85,29.26 C1.2 | 65.84,20.32 65.63,20.32 U1.8 | 65.84,20.32 66.85,20.32 C11.2 67.06,19.91 67.87,19.91 69.19,18.59 | 69.19,18.59 70.31,17.48 B1.P5-7 70.51,17.48 72.75,15.24 B1.P1-9 | 66.45,29.26 66.45,23.16 65.84,22.55 65.84,20.32 | 37.39,37.8 39.22,37.8 41.05,39.62 IC3.14 | 37.39,37.8 35.56,37.8 35.36,38 34.14,38 C4.2 | 37.39,48.77 39.01,48.77 41.05,50.8 IC2.14 | 37.39,48.77 35.76,48.77 35.56,48.97 34.14,48.97 C5.2 33.93,48.97 24.59,39.62 19.3,39.62 JP8.1 19.1,39.42 19.1,37.59 16.46,34.95 16.46,24.99 | 37.39,48.77 37.39,37.8 | 53.85,39.83 IC3.9 53.85,40.03 55.27,41.45 55.27,44.3 53.65,45.92 53.65,50.6 53.85,50.8 IC2.9 54.05,50.8 65.43,50.8 67.87,48.36 67.87,48.16 68.28,47.75 C3.2 | 69.19,18.59 70.31,19.71 B1.P5-8 | 16.46,24.99 13.82,24.99 U$15.K1
  Bottom 0.406: U$20.P$1 5,17.11 J1.SHUNT 3.76,9.96 3.86,9.96 | RESETA.1 13,77.18 13,71 6,71 U$1.P$1
  Bottom 0.508: 58.73,10.97 52.02,10.97 51.21,11.79 51.21,13.21 52.43,14.43 52.43,15.04 B1.P1-25 | 58.73,10.97 60.15,12.39 B1.P1-20 | 65.94,11.07 65.84,10.97 58.73,10.97 | 65.94,11.07 67.26,12.39 67.67,12.39 B1.P1-14 | B1.P1-6 77.83,12.39 77.42,12.39 76,10.97 66.04,10.97 65.94,11.07 | 92.35,79.35 94.89,81.89 GPIO3.1 | 92.35,79.35 86.56,73.56 81.48,73.56 SERIAL2.1 81.28,73.56 79.86,74.98 67.06,74.98 63.6,71.53 63.4,71.53 | 92.35,79.35 96.72,74.98 96.72,73.56 95.1,71.93 GPIO2.1 | 84.02,46.02 93.88,36.17 93.88,35.15 U$7.P$1 94.08,34.75 97.13,31.7 97.13,17.68 JOYSTICKS.8 | 84.02,46.02 77.62,52.43 UART1.5 | 84.02,46.02 94.89,56.9 94.89,61.57 GPIO1.1 | 54.05,52.83 54.05,51 IC2.9 | 54.05,52.83 54.05,59.13 57.51,62.59 57.51,63.2 B1.P6-1 57.71,63.4 57.71,64.62 63.4,70.31 63.4,71.53 | 63.4,71.53 61.98,72.95 61.98,73.36 SERIAL.1 | 54.05,52.83 43.08,52.83 41.25,51 IC2.14 | v64.21,31.7 61.98,31.7 54.05,39.62 IC3.9 | J1.GND 3.86,3.05 3.86,9.96 12.39,18.49 12.39,23.77 13.61,24.99 U$15.K1
  pour Top: 0,0 100,0 100,100 0,100
  pour Bottom: 0,0 100,0 100,100 0,100
GPA0  (via drill 0.41)
  Top 0.203: v67.87,38.81 68.68,39.62 68.68,40.03 U$23.4 | v56.9,38.2 55.07,38.2 54.46,37.59 51.61,37.59 50.39,38.81 50.39,40.84 51,41.45 51.61,41.45 52.83,42.67 52.83,49.38 51.41,50.8 IC2.10
  Bottom 0.203: v67.87,38.81 67.26,38.2 v56.9,38.2
GPA1  (via drill 0.41)
  Top 0.203: v65.23,42.47 68.48,42.47 69.29,41.66 69.29,40.23 U$23.5 | v58.73,42.47 54.25,38 53.03,38 51.41,39.62 IC3.10
  Bottom 0.203: v58.73,42.47 v65.23,42.47
GPA2  (via drill 0.41)
  Top 0.203: v96.32,55.68 80.87,40.23 80.87,31.09 80.06,30.28 78.84,30.28 78.03,31.09 78.03,32.11 77.42,32.72 76.61,32.72 70.1,39.22 70.1,40.03 U$23.6
  Bottom 0.203: v96.32,55.68 96.32,60.96 96.52,61.16 96.52,62.59 95.1,64.01 GPIO1.3
GPA3  (via drill 0.41)
  Top 0.203: v91.03,56.29 77.01,42.27 72.34,42.27 70.71,40.64 70.71,40.23 U$23.7
  Bottom 0.203: v91.03,56.29 91.03,62.59 92.46,64.01 GPIO1.4
GPA4
  Top 0.203: U$23.8 71.32,40.03 71.32,39.62 72.34,38.61 78.23,38.61 97.54,57.91 97.54,71.73 95.1,74.17 GPIO2.3
GPA5  (via drill 0.41)
  Top 0.203: v89.81,57.71 90.63,57.71 91.64,56.69 91.64,55.88 91.44,55.68 91.03,55.68 77.22,41.86 73.36,41.86 71.93,40.44 71.93,40.23 U$23.9
  Bottom 0.203: v89.81,57.71 89.81,71.53 92.46,74.17 GPIO2.4
GPA6  (via drill 0.41)
  Top 0.203: v90.42,54.05 77.83,41.45 73.56,41.45 72.75,40.64 72.75,40.23 U$23.10
  Bottom 0.203: v90.42,54.05 90.42,65.23 97.54,72.34 97.54,81.89 95.1,84.33 GPIO3.3
GPA7  (via drill 0.41)
  Top 0.203: v96.93,58.32 77.62,39.01 73.76,39.01 73.36,39.42 73.36,40.03 U$23.11
  Bottom 0.203: v96.93,58.32 96.93,61.16 97.94,62.18 97.94,83.52 95.71,85.75 93.88,85.75 92.66,84.53 GPIO3.4
GPB0  (via drill 0.41)
  Top 0.203: v73.97,44.7 73.97,45.72 U$23.13 | v81.89,26.82 89.81,18.9 90.02,18.9 90.83,18.09 90.83,16.26 89.61,15.04 JOYSTICKS.1
  Bottom 0.203: v73.97,44.7 82.09,36.58 82.09,27.03 v81.89,26.82
GPB1  (via drill 0.41)
  Top 0.203: v74.27,43.48 73.36,44.4 73.36,45.82 U$23.14 | v81.48,31.09 81.48,28.14 92.05,17.58 JOYSTICKS.4
  Bottom 0.203: v74.27,43.48 74.27,38.3 v81.48,31.09
MISO_3.3V  (via drill 0.41)
  Top 0.203: v57.71,18.09 57.71,20.32 U1.2
  Bottom 0.203: v57.71,18.09 57.71,15.24 B1.P1-21
MISO_5.0V  (via drill 0.41)
  Top 0.203: v42.88,38.2 42.67,38 42.67,31.29 50.19,23.77 56.69,23.77 58.93,21.54 58.93,20.52 U1.3
  Bottom 0.203: v42.88,38.2 42.88,38.61 42.67,38.81 42.67,40.84 | 42.67,40.84 43.28,41.45 44.5,41.45 46.13,39.83 IC3.12 | 42.67,40.84 42.67,44.09 46.13,47.55 46.13,50.8 IC2.12
MOSI_3.3V  (via drill 0.41)
  Top 0.203: v58.93,27.23 58.93,29.26 U3.3 | v54.86,23.16 54.86,19.91 59.54,15.24 60.15,15.24 B1.P1-19
  Bottom 0.203: v54.86,23.16 v58.93,27.23
MOSI_5.0V  (via drill 0.41)
  Top 0.203: v57.71,32.11 57.71,29.46 U3.2 | v55.07,35.97 53.85,37.19 51.41,37.19 48.97,39.62 IC3.11 48.77,39.83 47.75,40.84 47.75,44.09 48.77,45.11 48.77,50.8 IC2.11 48.77,51 48.77,59.94 40.44,68.28 v40.44,71.12 | v72.54,76 72.54,72.14 73.76,70.92 SERIAL2.8
  Bottom 0.203: v57.71,32.11 57.71,33.33 v55.07,35.97 | 54.25,71.53 54.25,71.73 55.47,72.95 55.47,75.59 61.57,81.69 65.43,81.69 71.12,76 v72.54,76 | 54.25,71.53 54.25,70.92 SERIAL.8 54.25,71.53 | v40.44,71.12 40.44,71.93 43.28,74.78 52.02,74.78 52.83,73.97 52.83,72.95 54.25,71.53
N$1  (via drill 0.41)
  Top 0.203: v66.85,39.01 66.85,40.03 U$23.1 | v64.62,39.01 64.62,39.42 64.01,40.03 R3.1
  Bottom 0.203: v64.62,39.01 v66.85,39.01
N$9
  Top 0.203: SJ2.2 84.53,52.43 82.7,52.43 UART1.9
N$10
  Top 0.203: SJ1.1 84.53,55.07 82.7,55.07 UART1.10
N$17
  Top 0.203: R8.1 18.49,22.96 14.22,22.96 13.82,22.55 U$15.A2
N$22  (via drill 0.41)
  Top 0.203: v17.27,27.03 18.49,27.03 R7.1
  Bottom 0.203: v17.27,27.03 14.22,27.03 13.82,27.43 U$15.A3
RESET
  Top 0.203: B1.P6-2 57.51,60.76 51.82,60.76 36.78,75.79 10.57,75.79 9.75,76.61 9.75,78.84 13.01,82.09 RESETA.3 13.21,82.3 15.85,82.3 RESETA1.3
RXD0_3.3V  (via drill 0.41)
  Top 0.203: v60.96,18.49 60.55,18.9 60.55,20.32 U1.4 | v61.98,17.48 61.98,16.05 61.37,15.44 v61.37,14.22
  Bottom 0.203: v61.98,17.48 v60.96,18.49 | v61.37,14.22 61.77,14.22 62.18,13.82 71.53,13.82 72.75,12.6 B1.P1-10
RXD0_5.0V  (via drill 0.41)
  Top 0.203: v44.91,44.91 44.91,30.68 51.41,24.18 58.52,24.18 61.57,21.13 61.57,20.52 U1.5 | v68.07,55.27 72.14,55.27 72.34,55.07 UART1.2
  Bottom 0.203: v44.91,44.91 45.31,44.91 49.38,48.97 57.51,48.97 61.98,53.44 66.24,53.44 v68.07,55.27
SCL_3.3V  (via drill 0.41)
  Top 0.203: 58.93,81.08 58.93,78.23 59.13,78.03 65.84,78.03 66.85,79.05 R1.1 | 58.93,81.08 58.93,81.48 60.76,83.31 62.18,83.31 63.8,81.69 63.8,81.08 Q2.2 | v40.23,10.16 74.78,10.16 76.61,11.99 76.61,13.01 77.83,14.22 77.83,15.04 B1.P1-5 | 58.93,81.08 v58.73,81.08
  Bottom 0.203: v40.23,10.16 16.87,33.53 16.87,49.58 48.36,81.08 v58.73,81.08
SCL_5.0V  (via drill 0.41)
  Top 0.203: v61.98,81.08 61.98,80.06 Q2.3 | 68.07,40.23 67.46,40.23 U$23.2 | 68.28,45.92 68.68,45.92 U$23.21 | 68.28,45.92 U$23.22 | v68.07,41.86 68.07,40.23 | 68.28,45.92 v68.28,44.3 | 68.07,40.23 U$23.3 | R9.1 76.2,79.05 76.2,75.39 77.62,73.97 77.62,72.14 78.84,70.92 SERIAL2.4 78.84,70.71 78.84,70.1 71.93,63.2 67.46,63.2 59.94,70.71 59.33,70.71 SERIAL.4
  Bottom 0.203: v61.98,81.08 61.98,77.83 57.91,73.76 57.91,72.14 59.13,70.92 SERIAL.4 | v68.07,41.86 68.07,42.27 68.48,42.67 68.48,44.09 v68.28,44.3 68.28,51.82 69.09,52.63 69.09,63.2 75.39,69.49 77.62,69.49 78.84,70.71 SERIAL2.4
SCLK_3.3V  (via drill 0.41)
  Top 0.203: v60.15,27.23 61.57,28.65 61.57,29.26 U3.5
  Bottom 0.203: v60.15,27.23 55.27,22.35 55.27,15.24 B1.P1-23
SCLK_5.0V  (via drill 0.41)
  Top 0.203: v73.76,77.22 73.76,73.56 SERIAL2.7 | v60.35,31.7 60.35,29.46 U3.4 | IC3.13 43.69,39.83 42.67,40.84 42.67,44.09 43.69,45.11 43.69,50.8 IC2.13 43.69,51 39.83,54.86 v39.83,70.31
  Bottom 0.203: 54.25,74.98 54.25,73.56 SERIAL.7 | 54.25,74.98 61.37,82.09 68.89,82.09 v73.76,77.22 | v60.35,31.7 54.05,38 45.52,38 43.89,39.62 IC3.13 | 54.25,74.98 52.43,74.98 52.22,75.18 43.08,75.18 39.83,71.93 v39.83,70.31
SDA_3.3V  (via drill 0.41)
  Top 0.203: v61.77,82.7 60.15,81.08 Q1.2 | v74.37,80.06 73.56,79.25 73.15,79.25 R4.1 | v91.24,80.06 98.55,72.75 98.55,14.43 93.07,8.94 86.97,8.94 85.95,9.96 85.95,11.58 83.72,13.82 82.5,13.82 81.28,15.04 80.67,15.04 B1.P1-3
  Bottom 0.203: v61.77,82.7 71.73,82.7 v74.37,80.06 v91.24,80.06
SDA_5.0V  (via drill 0.41)
  Top 0.203: 68.48,77.62 61.77,77.62 | 61.77,77.62 58.93,77.62 58.12,78.44 58.12,79.86 Q1.3 | 68.48,77.62 69.9,79.05 R2.1 | 61.77,77.62 v61.77,76 | v67.46,44.91 67.46,45.72 U$23.23 | v68.48,71.53 68.48,77.62
  Bottom 0.203: v61.77,76 59.33,73.56 SERIAL.3 | v67.46,44.91 67.46,51.61 68.68,52.83 68.68,64.01 72.34,67.67 | 72.34,67.67 75.18,70.51 75.18,71.53 75.79,72.14 77.62,72.14 78.84,73.36 SERIAL2.3 | 72.34,67.67 v68.48,71.53
TXD0_3.3V  (via drill 0.41)
  Top 0.203: v65.43,36.37 65.43,34.75 U3.9 | v68.28,36.37 69.29,36.37 v70.51,35.15
  Bottom 0.203: v68.28,36.37 v65.43,36.37 | v70.51,35.15 70.51,23.98 74.37,20.12 74.37,13.61 75.39,12.6 B1.P1-8
TXD0_5.0V  (via drill 0.41)
  Top 0.203: v62.99,49.17 62.99,39.62 64.01,38.61 64.01,34.75 U3.10 | v68.07,54.25 71.32,54.25 71.93,53.65 73.76,53.65 74.78,52.63 UART1.3
  Bottom 0.203: v68.07,54.25 v62.99,49.17
VIN  (via drill 0.61)
  Top 0.508: D1.C 22.35,10.16 22.35,13.82 IC1.3 22.55,13.82 v24.18,15.44 | 27.94,19.41 30.28,17.07 PC1.+ | 27.94,19.41 26.01,21.34 26.01,21.95 C2.1 | v27.84,19.1 27.84,19.3 27.94,19.41
  Bottom 0.508: v27.84,19.1 v24.18,15.44

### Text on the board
_tsilk: PCB-RPIBO1 | v10-13 | SKAARHOJ / 2013 | 5V | GND | 5V
_bsilk: GITHUB: SKAARHOJ-Open-Engineering

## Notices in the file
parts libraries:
SparkFun: Licensing: CC v3.0 Share-Alike You are welcome to use this library for commercial purposes.
